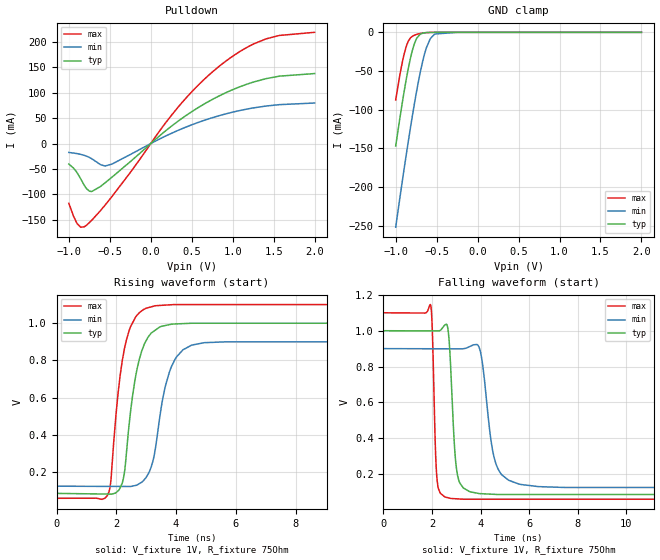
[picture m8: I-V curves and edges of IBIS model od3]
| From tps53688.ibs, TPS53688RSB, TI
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|   od3 Model
[Model]   od3
Model_type   Open_drain
Polarity   Non-Inverting
Vmeas = 0.5
Vref = 1
Cref = 2pF
Rref = 75
|   typ   min   max
C_comp   2.803pF   2.739pF   2.895pF
[Voltage Range]   1   0.9   1.1
|Junction Temperature
[Temperature Range]   25   125   -40
[Pullup Reference]   1   0.9   1.1
[Pulldown Reference]   0   0   0
[Power Clamp Reference]   1   0.9   1.1
[GND Clamp Reference]   0   0   0
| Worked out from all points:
|   slope of the pulldown table from 0 to 0.15 V, typ, clamps not added: 7.18 ohm
|   GND clamp passes 1 mA (typ) near -0.67 V on its own axis
|   falling waveform, V_fixture 1V, R_fixture 75Ohm: 20-80 % time 215ps typ, 442ps min, 125ps max; typ from 1 V to 0.086 V
|   rising waveform, V_fixture 1V, R_fixture 75Ohm: 20-80 % time 470ps typ, 540ps min, 442ps max; typ from 0.086 V to 1 V
[Pulldown]
|   Voltage   I(typ)   I(min)   I(max)
-1V       -40.23mA   -17.47mA   -117.3mA
-910mV    -54.78mA   -19.42mA   -154mA
-856mV    -69.06mA   -21.17mA   -164.4mA
-784mV    -88.51mA   -24.74mA   -160.5mA
-721mV    -94.27mA   -29.73mA   -150.9mA
-559mV    -77.41mA   -44.06mA   -121.3mA
-475mV    -66.31mA   -40.43mA   -104.5mA
296mV     39.51mA    23.31mA    64.2mA
794mV     90.34mA    52.9mA     146.5mA
1.094V    112.1mA    65.21mA    181.6mA
1.406V    127.6mA    73.79mA    205.8mA
2V        137.7mA    79.76mA    218.8mA
[GND Clamp]
|   Voltage   I(typ)   I(min)   I(max)
-1V       -146.9mA   -251.7mA   -87.48mA
-916mV    -88.68mA   -189.9mA   -37.03mA
-874mV    -62.43mA   -160.2mA   -19.24mA
-820mV    -33.52mA   -123.3mA   -7.237mA
-772mV    -14.86mA   -92.52mA   -3.763mA
-739mV    -7mA       -72.78mA   -2.536mA
-703mV    -2.686mA   -53.06mA   -1.569mA
-631mV    -399.9uA   -21.84mA   -443.1uA
-577mV    -105.8uA   -8.07mA    -130.2uA
-523mV    -27.93uA   -2.197mA   -32.17uA
-250mV    0A         -973.8nA   0A
2V        0A         0A         0A
[POWER Clamp]
|   Voltage   I(typ)   I(min)   I(max)
-1V       0A         0A         0A
2V        0A         0A         0A
[Ramp]
R_load = 75
|   typ   min   max
dV/dt_r   0.54854/4.68477e-10   0.465317/5.40186e-10   0.624273/4.415e-10
dV/dt_f   0.54854/2.14724e-10   0.465317/4.38389e-10   0.624273/1.23743e-10
[Falling Waveform]
V_fixture = 1V
V_fixture_min = 0.9V
V_fixture_max = 1.1V
R_fixture = 75Ohm
C_fixture = 0F
|   Time   V(typ)   V(min)   V(max)
0s        1V         900mV      1.1V
1.95ns    999mV      899.4mV    1.142V
2.195ns   998.8mV    899.3mV    191.6mV
2.621ns   1.032V     899.1mV    69.83mV
2.972ns   276.1mV    899mV      62.76mV
3.312ns   121.1mV    900mV      60.04mV
3.968ns   91.37mV    896.8mV    60.04mV
4.836ns   86.49mV    203.1mV    60.04mV
7.496ns   86.49mV    125.5mV    60.04mV
500ns     85.77mV    124.5mV    59.54mV
[Rising Waveform]
V_fixture = 1V
V_fixture_min = 0.9V
V_fixture_max = 1.1V
R_fixture = 75Ohm
C_fixture = 0F
|   Time   V(typ)   V(min)   V(max)
0s        85.77mV    124.5mV    59.54mV
1.708ns   82.2mV     123.4mV    76.05mV
1.812ns   81.98mV    123.3mV    144.8mV
2.103ns   107mV      123.1mV    682.7mV
2.433ns   458.8mV    122.9mV    960.9mV
2.851ns   849.8mV    145.8mV    1.066V
3.223ns   953mV      257.3mV    1.09V
3.918ns   995.1mV    789.6mV    1.099V
5.675ns   999.6mV    899.5mV    1.099V
500ns     1V         900mV      1.1V
